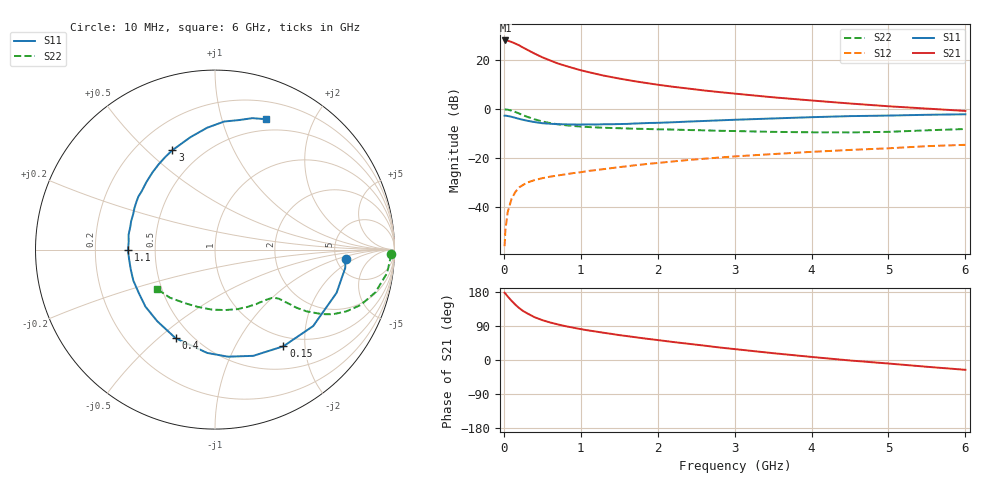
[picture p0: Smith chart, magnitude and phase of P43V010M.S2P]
! SIEMENS Small Signal Semiconductors
! BFP182
! Si NPN RF Bipolar Junction Transistor in SOT143
! VCE = 3 V  IC = 10 mA
! Common Emitter S-Parameters:  March  1996
# GHz  S  MA  R  50
!  f  S11  S21  S12  S22
! GHz  MAG  ANG  MAG  ANG  MAG  ANG  MAG  ANG
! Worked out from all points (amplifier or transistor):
!   36 points, 10 MHz to 6 GHz, reference 50 ohm
!   highest |S21| = 27.9 dB at 20 MHz (marker M1)
!   |S21| within 3 dB of that: start of sweep to 255.8 MHz
!   unconditionally stable (mu >= 1): 1.162 GHz to 5.392 GHz
!   at 250 MHz: K = 0.33, MSG = 28.0 dB, |S12| = -31.0 dB
!   at 1.4 GHz: K = 1.08, MAG = 16.8 dB, |S12| = -24.1 dB
!   at 6 GHz: K = 0.94, MSG = 6.9 dB, |S12| = -14.6 dB
!   lowest NFmin = 1.50 dB at 450 MHz
!   S11 on the Smith chart (normalised r, x): 10 MHz: 6.09, -1.32; 150 MHz: 0.84, -1.60; 400 MHz: 0.41, -0.57; 1.1 GHz: 0.35, -0.00; 3 GHz: 0.35, +0.60; 6 GHz: 0.38, +1.40
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0.01  0.729 -4.0  24.89 177.4  0.0016 91.8  0.9822 -1.5
0.02  0.7328 -8.0  24.92 175.3  0.0034 88.8  0.9777 -3.1
0.05  0.7189 -19.6  24.66 167.7  0.0079 81.4  0.9679 -7.7
0.1  0.6932 -37.9  23.19 156.3  0.0147 72.6  0.925 -14.9
0.15  0.6598 -54.7  21.5 145.9  0.0204 63.9  0.8688 -20.8
0.2  0.6291 -70.2  19.79 136.9  0.0253 60.0  0.8073 -25.3
0.25  0.6009 -83.1  17.84 129.4  0.0283 54.9  0.7481 -28.8
0.3  0.5775 -94.3  16.22 123.5  0.0315 52.5  0.6961 -31.1
0.4  0.5404 -113.9  13.44 112.9  0.0355 47.9  0.6153 -34.0
0.5  0.5126 -128.9  11.31 105.2  0.0389 45.3  0.5571 -35.5
0.6  0.5011 -140.7  9.786 99.1  0.0417 44.1  0.5167 -36.1
0.7  0.4886 -150.4  8.489 94.0  0.0441 44.0  0.4888 -36.7
0.9  0.4822 -166.6  6.823 85.4  0.0493 44.1  0.4509 -37.5
1.1  0.485 -179.5  5.648 78.0  0.0546 44.5  0.4288 -39.0
1.5  0.4931 161.4  4.173 65.7  0.0653 44.9  0.4055 -42.8
1.8  0.5122 148.8  3.48 57.6  0.0738 44.7  0.3934 -46.7
2.2  0.5362 135.5  2.836 47.5  0.0853 43.2  0.3806 -53.1
3  0.6025 113.2  2.058 28.8  0.108 38.6  0.3552 -68.9
3.5  0.6409 102.4  1.73 18.0  0.1205 34.9  0.3416 -80.5
4.5  0.7154 85.9  1.293 -1.3  0.1463 27.6  0.3332 -106.7
5.5  0.7615 74.1  1.018 -17.9  0.1747 20.3  0.3676 -133.3
6  0.7801 68.6  0.913 -25.9  0.1861 15.6  0.3908 -146.0
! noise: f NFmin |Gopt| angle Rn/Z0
0.45  1.5  0.26  43  0.28
0.9  1.6  0.24  87  0.22
1.8  2.1  0.2  170  0.2
